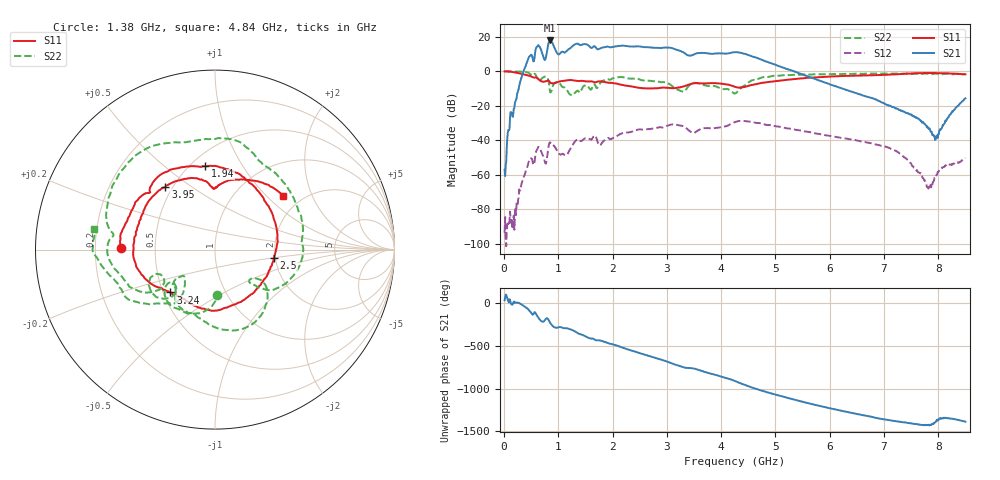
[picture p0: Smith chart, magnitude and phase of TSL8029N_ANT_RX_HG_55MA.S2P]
!Agilent Technologies,E5071C,MY46523237,B.13.01
!Date: Wed Oct 18 11:28:39 2023
!Data & Calibration Information:
!Freq	S11:SOLT2(ON)	S21:SOLT2(ON)	S12:SOLT2(ON)	S22:SOLT2(ON)
!PortZ  Port1:50+j0  Port2:50+j0
!Above PortZ is port z conversion or system Z0 setting when saving the data.
!When reading, reference impedance value at option line is always used.
# Hz S dB R 50
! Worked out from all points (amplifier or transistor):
!   850 points, 10 MHz to 8.5 GHz, reference 50 ohm
!   highest |S21| = 17.9 dB at 840 MHz (marker M1)
!   |S21| within 3 dB of that: 1.273 GHz to 1.558 GHz (285.4 MHz wide, 20.2 % of centre)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
!   unconditionally stable (mu >= 1): 30 MHz to 47.14 MHz; 73.5 MHz to end of sweep
!   at 1.42 GHz: K = 6.18, MAG = 17.0 dB, |S12| = -40.4 dB
!   at 4.26 GHz: K = 3.33, MAG = 12.1 dB, |S12| = -29.3 dB
!   at 8.5 GHz: K = 93.84, MAG = -5.5 dB, |S12| = -50.1 dB
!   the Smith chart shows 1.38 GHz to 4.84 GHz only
!   S11 on the Smith chart (normalised r, x): 1.38 GHz: 0.31, +0.01; 1.94 GHz: 0.59, +0.70; 2.5 GHz: 1.96, -0.20; 3.24 GHz: 0.55, -0.30; 3.95 GHz: 0.46, +0.40; 4.84 GHz: 1.61, +1.26
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1e7  0.00 -2.0  -57.05 34.9  -93.62 26.3  0.03 -1.8
4.1e8  -2.12 -74.0  4.33 -52.4  -56.47 174.2  -0.42 -84.2
5.9e8  -3.56 -100.9  13.61 -128.0  -46.56 109.6  -2.52 -129.8
6.9e8  -5.75 -111.4  11.73 148.6  -46.88 29.3  -4.27 -125.4
7.9e8  -5.51 -115.1  11.30 -176.6  -50.39 70.0  -3.31 -165.9
8.4e8  -6.09 -127.1  17.94 140.2  -41.25 36.0  -10.40 170.1
9.4e8  -6.73 -125.0  12.99 74.8  -44.01 -25.1  -6.51 -160.4
1.26e9  -5.09 -165.9  14.61 45.1  -42.73 -25.9  -13.73 20.1
1.38e9  -5.63 179.1  15.64 1.0  -39.58 -71.0  -11.91 -87.1
1.43e9  -5.47 172.2  15.37 -7.4  -40.25 -77.0  -10.39 -91.5
1.55e9  -5.80 156.4  15.13 -45.0  -38.99 -108.8  -8.86 -141.3
1.94e9  -6.60 96.9  14.10 -112.8  -39.03 -165.7  -4.86 172.3
2.22e9  -8.11 46.3  14.86 -168.9  -35.52 152.7  -3.56 117.9
2.5e9  -9.59 -7.9  14.44 135.0  -33.58 99.5  -4.71 69.5
2.84e9  -9.73 -75.2  13.63 69.5  -32.52 39.2  -5.90 15.5
3.24e9  -9.26 -136.1  11.94 -16.6  -31.32 -48.1  -11.14 -43.6
3.95e9  -7.00 128.2  10.46 -129.8  -32.55 -146.8  -9.29 -130.3
4.26e9  -9.01 93.6  11.16 167.5  -29.31 163.4  -12.77 -137.5
4.84e9  -6.30 38.4  5.62 38.3  -31.02 35.1  -3.33 170.5
5.67e9  -3.57 -76.7  -3.70 -101.5  -35.50 -104.9  -1.83 46.7
7.09e9  -1.90 144.7  -19.92 70.9  -44.28 33.5  -1.27 -135.0
8.5e9  -1.69 -20.9  -15.63 52.2  -50.12 31.8  -1.56 71.0
